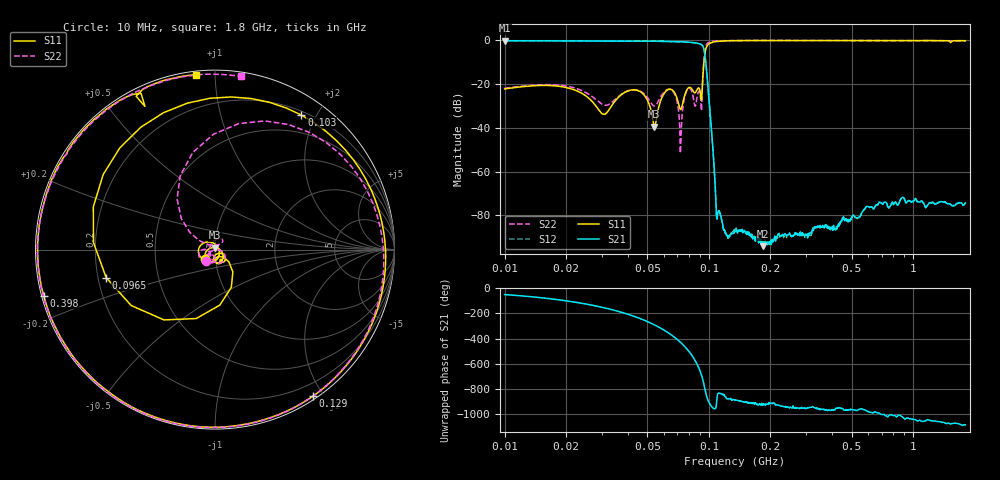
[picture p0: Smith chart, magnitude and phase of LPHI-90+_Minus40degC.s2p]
! Mini-Circuits
! S2P DATA File Format
! Type:LOW PASS FILTER
! Model: LPHI-90+
! All S Parameters are in dB deg format
! TEST CONDITIONS: INPUT POWER = 0 dBm,  -40deg C
# MHz S DB R 50
!Frequency  S11 dB  S11 DEG  S21 dB  S21 DEG  S12 dB  S12 DEG  S22 dB  S22 DEG
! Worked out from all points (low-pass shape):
!   493 points, 10 MHz to 1.8 GHz, reference 50 ohm
!   highest |S21| = -0.16 dB at 10 MHz (marker M1); lowest = -94.0 dB at 184 MHz (marker M2)
!   |S21| within 3 dB of the highest: start of sweep to 93.9 MHz
!   lowest |S11| = -39.4 dB at 54 MHz (marker M3), VSWR 1.02, Z = 49.9 + j1.07 ohm
!   |S11| at or under -10 dB: start of sweep to 94.54 MHz
!   |S22| runs from -51.6 to 0.0 dB; largest |S21 - S12| = 0.0009
!   S11 on the Smith chart (normalised r, x): 10 MHz: 0.89, -0.10; 96.5 MHz: 0.23, -0.12; 103 MHz: 0.25, +1.80; 129 MHz: 0.04, -1.88; 398 MHz: 0.01, -0.13; 1.8 GHz: 0.02, +0.90
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10  -22.16 -136.1  -0.16 -49.9  -0.16 -49.9  -21.90 -126.7
24  -24.31 135.8  -0.23 -120.2  -0.23 -120.2  -23.03 -179.2
38  -24.26 -87.2  -0.30 165.0  -0.29 165.0  -24.12 -121.3
54  -39.38 94.1  -0.40 69.5  -0.39 69.5  -29.99 -119.0
56.5  -31.38 -1.9  -0.42 53.0  -0.42 53.0  -27.82 -93.7
67  -23.16 -87.6  -0.56 -23.2  -0.55 -23.2  -23.54 -126.9
72.5  -31.53 -71.0  -0.64 -69.6  -0.63 -69.6  -51.58 -138.2
76.5  -24.42 -32.2  -0.74 -107.5  -0.74 -107.5  -25.00 -24.4
82  -21.92 -62.8  -0.94 -167.8  -0.94 -167.8  -22.88 -85.2
88.5  -21.79 -65.6  -1.39 99.1  -1.38 99.1  -23.88 72.5
92.5  -24.06 -42.2  -2.16 15.6  -2.16 15.6  -25.62 145.3
96.5  -4.07 -165.6  -9.99 -112.6  -9.99 -112.7  -2.92 79.3
99.5  -1.78 110.5  -24.08 -179.9  -24.09 -179.9  -1.01 31.4
103  -1.00 57.3  -41.37 138.8  -41.38 138.8  -0.57 1.2
109.5  -0.49 5.8  -81.58 -148.0  -81.54 -149.8  -0.29 -30.9
129  -0.16 -56.1  -88.56 -171.5  -87.78 -164.7  -0.10 -76.0
135  -0.13 -66.4  -86.64 -167.5  -87.66 -171.0  -0.09 -84.3
184  -0.08 -111.6  -94.03 161.5  -92.04 149.4  -0.04 -122.5
320  -0.10 -153.9  -86.66 137.4  -87.35 136.8  -0.08 -159.9
398  -0.10 -165.0  -86.12 108.3  -85.39 105.3  -0.08 -169.7
760  -0.11 164.9  -76.64 66.2  -76.40 67.0  -0.12 160.3
1800  -0.16 96.3  -74.28 -7.9  -74.35 -9.2  -0.22 81.5
